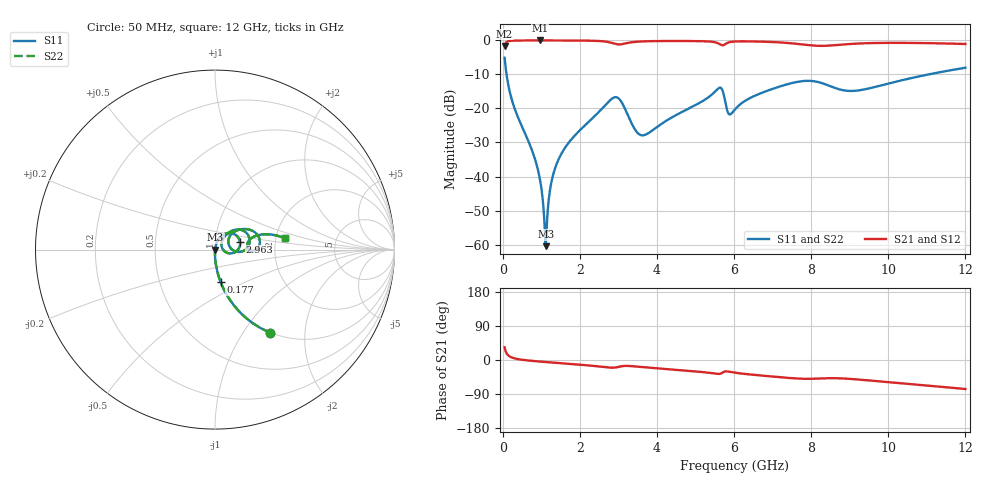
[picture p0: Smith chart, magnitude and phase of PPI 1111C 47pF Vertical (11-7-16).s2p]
# GHz S MA R 50
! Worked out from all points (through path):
!   1601 points, 50 MHz to 12 GHz, reference 50 ohm
!   highest |S21| = -0.01 dB at 968.7 MHz (marker M1); lowest = -1.6 dB at 50 MHz (marker M2)
!   group delay of S21, straight-line fit = 17.5 ps
!   lowest |S11| = -60.5 dB at 1.118 GHz (marker M3), VSWR 1.00, Z = 50.1 + j0.00937 ohm
!   |S11| at or under -10 dB: 100.1 MHz to 11.04 GHz (10.94 GHz wide, 196 % of centre)
!   |S22| runs from -60.5 to -5.1 dB; largest |S21 - S12| = 0
!   S11 on the Smith chart (normalised r, x): 50 MHz: 0.99, -1.34; 177 MHz: 1.00, -0.37; 2.963 GHz: 1.32, +0.11; 12 GHz: 2.26, +0.33
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0.05  0.557 -56.4  0.8303 33.6  0.8303 33.6  0.557 -56.4
0.1769688  0.1822 -80.2  0.9828 9.6  0.9828 9.6  0.1822 -80.2
0.8043438  0.02064 -90.6  0.999 -2.7  0.999 -2.7  0.02064 -90.6
0.9686562  0.008925 -88.8  0.9991 -4.2  0.9991 -4.2  0.008925 -88.8
1.073219  0.002587 -74.7  0.999 -5.0  0.999 -5.0  0.002587 -74.7
1.118031  0.0009463 5.7  0.999 -5.4  0.999 -5.4  0.0009463 5.7
1.155375  0.002486 61.7  0.999 -5.7  0.999 -5.7  0.002486 61.7
1.252469  0.007667 75.8  0.9989 -6.5  0.9989 -6.5  0.007667 75.8
1.386906  0.01467 77.9  0.9986 -7.5  0.9986 -7.5  0.01467 77.9
2.044156  0.05047 73.4  0.9952 -12.7  0.9952 -12.7  0.05047 73.4
2.962813  0.1457 17.0  0.8785 -19.1  0.8785 -19.1  0.1457 17.0
3.537906  0.04182 6.5  0.9616 -17.9  0.9616 -17.9  0.04182 6.5
4.038312  0.05524 47.2  0.979 -22.2  0.979 -22.2  0.05524 47.2
5.614219  0.2006 25.3  0.8898 -36.7  0.8898 -36.7  0.2006 25.3
5.696375  0.1868 5.5  0.8477 -33.6  0.8477 -33.6  0.1868 5.5
5.868156  0.08259 13.1  0.9386 -30.9  0.9386 -30.9  0.08259 13.1
6.025  0.09685 38.1  0.965 -33.6  0.965 -33.6  0.09685 38.1
6.839094  0.1801 38.6  0.9548 -42.2  0.9548 -42.2  0.1801 38.6
8.019156  0.2534 9.1  0.844 -49.6  0.844 -49.6  0.2534 9.1
8.997563  0.1809 5.8  0.8861 -49.8  0.8861 -49.8  0.1809 5.8
10.01331  0.2331 18.5  0.921 -58.5  0.921 -58.5  0.2331 18.5
12  0.3971 9.0  0.8868 -76.5  0.8868 -76.5  0.3971 9.0
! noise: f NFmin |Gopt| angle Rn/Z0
0.05  0.0003589  0.8617  0.6689  0.0005563
1.372  0.00388  0.6829  6.557  0.002363
2.701  0.03177  0.914  12.94  0.08034
4.031  0.02707  0.8558  19.18  0.03899
5.36  0.03578  0.8573  25.23  0.05106
6.682  0.03933  0.8427  31.12  0.04925
8.012  0.1029  0.9265  37  0.2793
9.341  0.08184  0.8968  42.57  0.1504
10.67  0.06176  0.852  47.79  0.07448
12  0.05724  0.8286  52.74  0.05655
